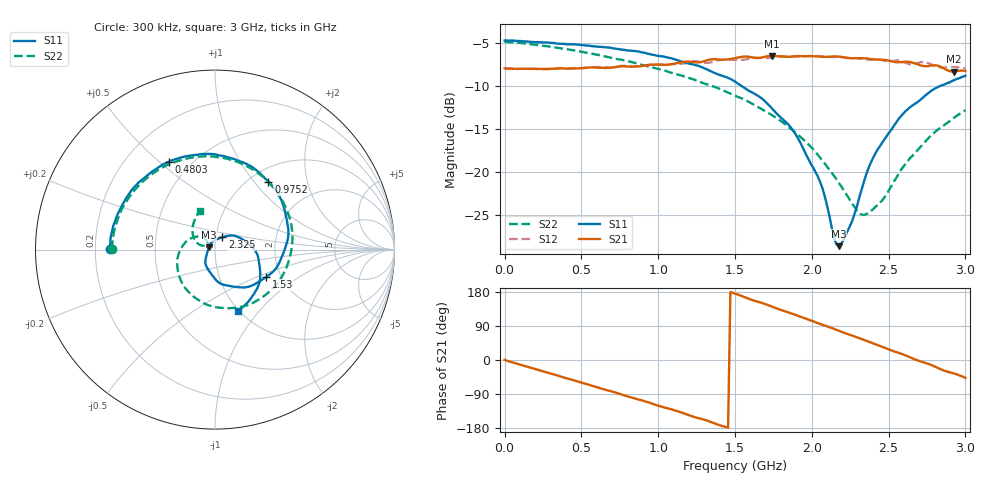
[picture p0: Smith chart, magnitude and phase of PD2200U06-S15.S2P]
!Agilent Technologies,E5071B,MY42302032,A.08.01
!Date: Sat Mar 25 16:44:02 2017
!Data & Calibration Information:
!Freq	S11:SOLT2(ON)	S21:SOLT2(ON)	S12:SOLT2(ON)	S22:SOLT2(ON)
# Hz S dB R 50
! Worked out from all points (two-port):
!   201 points, 300 kHz to 3 GHz, reference 50 ohm
!   highest |S21| = -6.44 dB at 1.74 GHz (marker M1); lowest = -8.3 dB at 2.925 GHz (marker M2)
!   |S21| within 3 dB of the highest: start of sweep to end of sweep
!   lowest |S11| = -28.6 dB at 2.175 GHz (marker M3), VSWR 1.08, Z = 46.6 + j1.23 ohm
!   |S11| at or under -10 dB: 1.545 GHz to 2.83 GHz (1.285 GHz wide, 58.7 % of centre)
!   |S22| runs from -25.0 to -4.8 dB; largest |S21 - S12| = 0.029
!   S11 on the Smith chart (normalised r, x): 300 kHz: 0.26, +0.00; 480.3 MHz: 0.38, +0.54; 975.2 MHz: 1.21, +1.19; 1.53 GHz: 1.67, -0.57; 2.325 GHz: 1.07, +0.15; 3 GHz: 0.99, -0.78
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300000  -4.65 179.8  -7.90 0.2  -7.90 0.3  -4.81 179.7
1.20288e8  -4.75 163.9  -7.97 -14.5  -7.93 -14.5  -4.97 153.6
2.552745e8  -4.88 146.5  -7.98 -30.4  -7.97 -30.6  -5.28 125.0
4.80252e8  -5.13 117.7  -7.90 -57.1  -7.89 -57.2  -5.90 78.8
5.10249e8  -5.19 113.9  -7.87 -60.7  -7.87 -60.7  -6.00 72.8
7.50225e8  -5.69 82.4  -7.67 -89.5  -7.64 -89.4  -6.87 25.0
9.752025e8  -6.35 51.8  -7.46 -117.3  -7.46 -117.3  -7.85 -19.0
1.0052e9  -6.46 47.5  -7.47 -121.1  -7.44 -121.4  -7.99 -24.7
1.230177e9  -7.45 15.5  -7.14 -149.8  -7.08 -149.5  -9.19 -68.4
1.50015e9  -9.44 -23.8  -6.72 175.5  -6.90 174.5  -11.09 -121.0
1.530147e9  -9.81 -28.2  -6.61 171.2  -6.91 170.6  -11.30 -126.9
1.740126e9  -12.57 -61.9  -6.44 140.8  -6.66 142.2  -13.35 -166.5
1.875112e9  -15.07 -86.1  -6.53 121.7  -6.50 122.0  -15.13 169.6
2.010099e9  -19.52 -116.9  -6.49 101.9  -6.44 102.3  -17.35 149.2
2.175082e9  -28.65 159.2  -6.53 77.4  -6.59 78.0  -21.25 132.1
2.265074e9  -25.59 89.7  -6.71 64.1  -6.71 64.5  -23.75 132.9
2.325068e9  -21.99 59.1  -6.71 55.2  -6.77 55.5  -24.96 140.9
2.40006e9  -18.30 40.3  -6.85 43.6  -6.90 44.9  -24.32 155.2
2.50505e9  -15.37 17.0  -7.00 27.4  -7.08 29.2  -22.04 163.2
2.730027e9  -11.22 -24.3  -7.63 -6.4  -7.16 -5.2  -16.62 146.6
2.925008e9  -9.28 -56.9  -8.27 -35.3  -7.71 -34.9  -13.67 121.8
3e9  -8.77 -69.3  -8.20 -47.0  -7.90 -47.0  -12.78 111.4
